(* Logix 5000 AddOnInstructionDefinition export ACS_SET_DIGITAL_OUTPUTS; software revision 24.00 *)

ADD_ON_INSTRUCTION ACS_SET_DIGITAL_OUTPUTS   (* revision 2.1, vendor Tolomatic, Inc *)
// Set Digital Output Bits on ACS Drive and Controller
VAR_IN_OUT
   DriveDigitalOutput : DINT; {required}   // ACS.0.DIGITAL_OUTPUT
END_VAR
VAR_INPUT
   DigitalOutput1 : BOOL; {visible}   // Digital Output 1
   DigitalOutput2 : BOOL; {visible}   // Digital Output 2
   DigitalOutput3 : BOOL; {visible}   // Digital Output 3
   DigitalOutput4 : BOOL; {visible}   // Digital Output 4
   DigitalOutputBrake : BOOL; {visible}   // Digital Output Brake Enable (Only valid if Brake is not configured on Drive. If Brake is configured, it is controlled automatically by drive using motor Enable/Disable
END_VAR
VAR
   DigitalOutputs : DINT; {access None}   // Combined value of the digital inputs
END_VAR

ROUTINE Logic   (* ladder *)
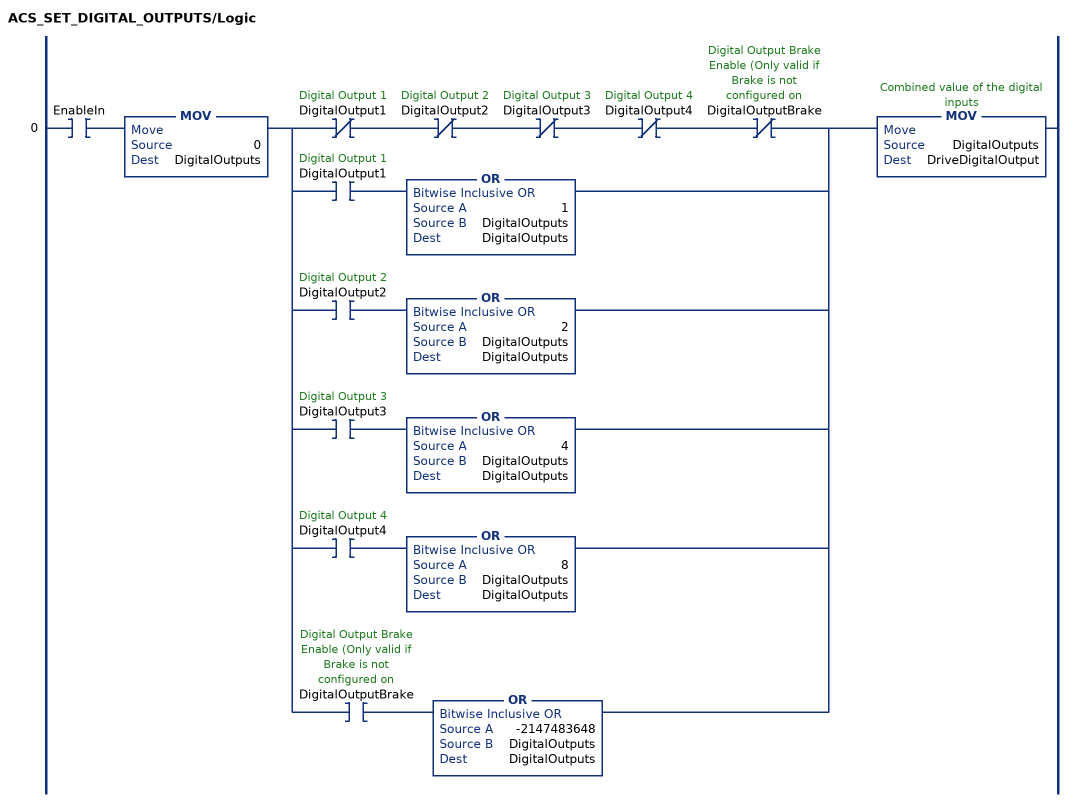
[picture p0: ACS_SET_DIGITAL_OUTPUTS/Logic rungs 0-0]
   0: XIC(EnableIn)MOV(0,DigitalOutputs)[XIO(DigitalOutput1) XIO(DigitalOutput2) XIO(DigitalOutput3) XIO(DigitalOutput4) XIO(DigitalOutputBrake) ,XIC(DigitalOutput1) OR(1,DigitalOutputs,DigitalOutputs) ,XIC(DigitalOutput2) OR(2,DigitalOutputs,DigitalOutputs) ,XIC(DigitalOutput3) OR(4,DigitalOutputs,DigitalOutputs) ,XIC(DigitalOutput4) OR(8,DigitalOutputs,DigitalOutputs) ,XIC(DigitalOutputBrake) OR(-2147483648,DigitalOutputs,DigitalOutputs) ]MOV(DigitalOutputs,DriveDigitalOutput);
END_ROUTINE
END_ADD_ON_INSTRUCTION
